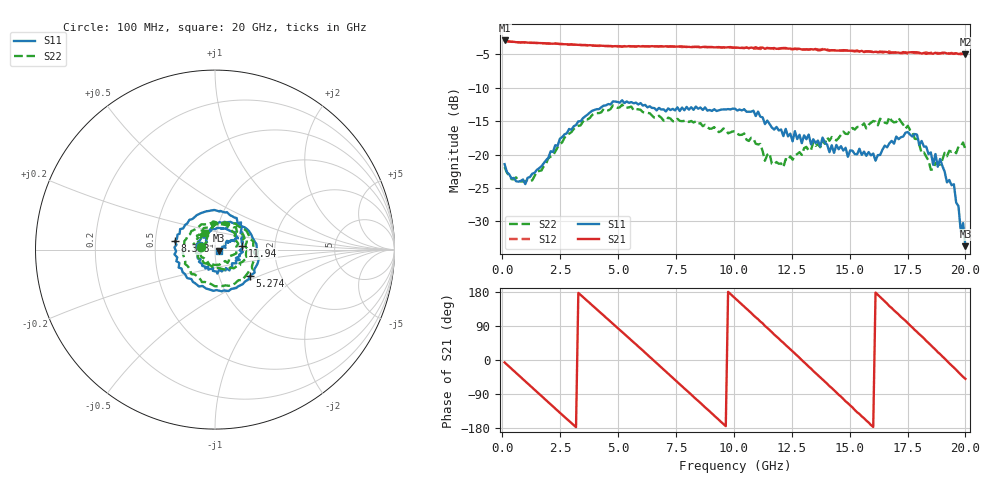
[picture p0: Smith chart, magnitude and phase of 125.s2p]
!Agilent Technologies,N5230C,MY49001569,A.09.33.09
!Agilent N5230C: A.09.33.09
!Date: Tuesday, July 28, 2015 11:15:56
!Correction: S11(Full 2 Port(1,2))
!S21(Full 2 Port(1,2))
!S12(Full 2 Port(1,2))
!S22(Full 2 Port(1,2))
!S2P File: Measurements: S11, S21, S12, S22:
# Hz S  dB  R 50
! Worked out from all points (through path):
!   201 points, 100 MHz to 20 GHz, reference 50 ohm
!   highest |S21| = -2.91 dB at 100 MHz (marker M1); lowest = -5.0 dB at 20 GHz (marker M2)
!   group delay of S21, straight-line fit = 156 ps
!   lowest |S11| = -33.7 dB at 20 GHz (marker M3), VSWR 1.04, Z = 52 - j0.692 ohm
!   |S11| at or under -10 dB: start of sweep to end of sweep
!   |S22| runs from -24.0 to -12.5 dB; largest |S21 - S12| = 0.023
!   S11 on the Smith chart (normalised r, x): 100 MHz: 0.85, +0.03; 5.274 GHz: 1.39, -0.44; 8.358 GHz: 0.63, +0.06; 11.94 GHz: 1.35, +0.06; 20 GHz: 1.04, -0.01
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1e8  -21.43 167.7  -2.91 -6.5  -2.93 -6.3  -21.87 170.1
9.955e8  -24.42 137.9  -3.19 -56.3  -3.24 -56.4  -24.04 138.9
1.7915e9  -21.28 121.9  -3.32 -100.6  -3.31 -100.5  -21.72 122.3
2.687e9  -16.97 88.1  -3.46 -150.2  -3.49 -150.0  -17.47 92.0
3.483e9  -14.55 50.2  -3.59 166.1  -3.61 165.9  -15.05 55.5
4.3785e9  -12.67 7.8  -3.72 117.4  -3.76 117.2  -13.16 11.5
5.274e9  -12.28 -37.7  -3.77 68.6  -3.75 68.3  -12.97 -32.0
6.7665e9  -13.00 -113.4  -3.81 -13.8  -3.79 -14.2  -14.19 -112.0
8.3585e9  -12.81 168.0  -3.88 -102.7  -3.88 -102.9  -15.03 164.7
9.254e9  -13.47 126.8  -3.93 -152.2  -3.90 -152.3  -16.30 113.7
1.005e10  -13.13 90.6  -3.97 163.1  -4.00 162.8  -16.54 62.9
1.09455e10  -14.22 49.2  -3.92 112.6  -4.13 112.3  -18.38 8.3
1.19405e10  -16.38 8.1  -4.13 56.6  -4.18 55.6  -21.38 -81.9
1.27365e10  -17.68 -27.3  -4.15 11.4  -4.25 10.3  -19.92 -148.3
1.3433e10  -17.70 -63.0  -4.27 -29.0  -4.20 -29.2  -18.10 166.9
1.47265e10  -19.40 -131.1  -4.36 -102.6  -4.47 -102.7  -16.56 88.9
1.5821e10  -19.62 156.1  -4.53 -164.9  -4.58 -165.7  -15.53 35.7
1.67165e10  -18.32 85.2  -4.79 142.2  -4.55 142.2  -14.35 -0.1
1.79105e10  -17.02 32.1  -4.68 74.1  -4.80 73.4  -17.71 -59.1
1.9005e10  -21.69 36.4  -4.75 9.5  -4.79 9.0  -20.76 178.3
1.95025e10  -24.44 9.6  -4.89 -20.0  -4.93 -20.5  -19.45 144.2
2e10  -33.71 -18.8  -4.99 -49.7  -4.93 -50.3  -19.23 119.4
